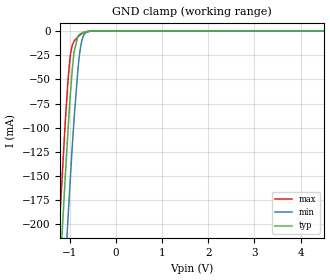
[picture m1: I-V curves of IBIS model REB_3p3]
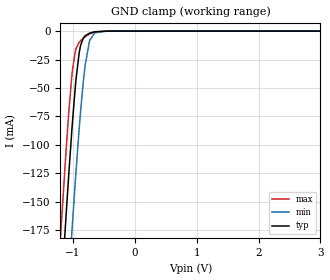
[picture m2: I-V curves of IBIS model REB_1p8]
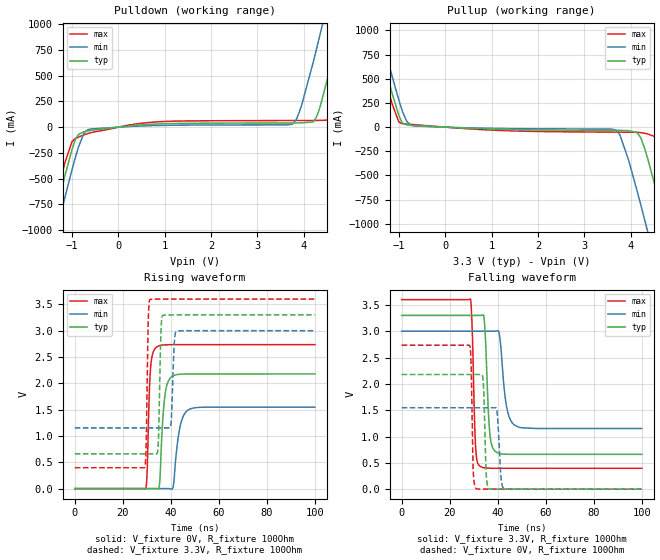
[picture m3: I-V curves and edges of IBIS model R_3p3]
|Texas Instruments Incorporated
| 3.3V RS-485 with flexible I/O supply and selectable speed
| Marketing part#   Digital Voltage Range   Package-type   #pins
| SN65HVD01   1.62V - 3.6V   VSON   10
[IBIS Ver]   4.1
[File name]   sn65hvd01.ibs
[File Rev]   1.1
[Date]   10/19/2016
[Source]
| Texas Instruments Incorporated.
| Analog-eLab Design Center, HPA
| 12500 TI Blvd
| Dallas, TX -75243
[Notes]   Revision History:
| Rev 1.2:10/19/2016
| - 2.5V model added for REB_xxx, R_xxx and DE_xxx.
|   Model names with a trailing _2p5 contains the model for
|   2.5V operation
| Rev 1.1: 04/09/2015
| - AB_ls model has been updated to better reflect the driver behavior.
| Rev 1.0: 05/08/2013
| - Initial version of the model
| - Model generated from simulations in TISPICE
| - C_comp although listed in numerical order of value are
|   obtained from varying PVT conditions. For PVT conditions for
|   each specific value refer the buffer description under
|   respective [Model]. IBIS model user is responsible for using
|   appropriate C_comp to simulate for Signal Integrity.
| - Warnings regarding combined Non-monotonicity of various models have been
|   reviewd and considered minor and can be ignored.
| - Model names with a trailing _1p8 contains the model for
|   1.8V operation.Model names with a trailing _3p3 contains the model
|   for 3.3V operation.
| - Mode names with a trailing _ls and _hs are for low speed and high speed
|   buffer operation, respectively.
[Disclaimer]
| This model is designed as an aid for customers of Texas Instruments.
| TI and its licensors and suppliers make no warranties, either expressed
| or implied, with respect to this  model, including the warranties of
| merchantability or fitness for a particular purpose. The model is
| provided solely on an "as is" basis. The entire risk as to its quality
| and performance is with the customer.
[Copyright]
 (C) Copyright 2013 Texas Instruments Incorporated.All rights reserved.
|   SN65HVD01
[Component]   SN65HVD01
[Manufacturer]   TI
[Package]   | 10 PIN VSON
|   typ   min   max
R_pkg   0.067   0.027   0.083
L_pkg   0.937nH   0.593nH   1.143nH
C_pkg   0.144pF   0.126pF   0.200pF
[Pin]  signal_name   model_name   R_pin   L_pin   C_pin
1   VL   POWER   NA   NA   NA
2   R   R   NA   NA   NA
3   DE   DE   NA   NA   NA
4   REB   REB   NA   NA   NA
5   D   REB   NA   NA   NA
6   GND   GND   NA   NA   NA
7   SLR   DE   NA   NA   NA
8   A   AB   NA   NA   NA
9   B   AB   NA   NA   NA
10   VCC   POWER   NA   NA   NA
[Diff Pin]  inv_pin  vdiff  tdelay_typ tdelay_min tdelay_max
8   9   200mV   NA   NA   NA
|   Model Selectors
[Model Selector]  DE
DE_3p3   DE buffer in 3.3V operation
DE_1p8   DE buffer in 1.8V operation
DE_2p5   DE buffer in 2.5V operation
[Model Selector]  REB
REB_3p3   REB buffer in 3.3V operation
REB_1p8   REB buffer in 1.8V operation
REB_2p5   REB buffer in 2.5V operation
[Model Selector]  R
R_3p3   R buffer in 3.3V operation
R_1p8   R buffer in 1.8V operation
R_2p5   R buffer in 2.5V operation
[Model Selector]  AB
AB_hs   high speed AB buffer operation
AB_ls   low speed AB buffer operation
| Models and submodels in the file (11): REB_3p3 (Input), REB_1p8 (Input), R_3p3 (Output), R_1p8 (Output), DE_3p3 (Input), DE_1p8 (Input), AB_ls (I/O), AB_hs (I/O), REB_2p5 (Input), R_2p5 (Output), DE_2p5 (Input)
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|   Model
[Model]   REB_3p3
Model_type   Input
Vinl = 0.99
Vinh = 2.31
|   typ   min   max
C_comp   0.767pF   0.735pF   0.817pF
[Voltage Range]   3.3   3   3.6
[Temperature Range]   27   125   -40
[Power Clamp Reference]   3.3   3   3.6
[GND Clamp Reference]   -0   -0   -0
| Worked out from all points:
|   GND clamp passes 1 mA (typ) near -0.68 V on its own axis
[GND Clamp]
|   Voltage   I(typ)   I(min)   I(max)
-3.3V     -2.277A    -2.364A    -2.225A
-1.231V   -268.8mA   -364.6mA   -209.6mA
-1.211V   -251mA     -346.7mA   -191.9mA
-1.092V   -147.7mA   -241.5mA   -91.49mA
-1.043V   -107.7mA   -199.2mA   -55.66mA
-983.4mV  -64.12mA   -150.4mA   -24.67mA
-914.1mV  -25.42mA   -97.58mA   -11.23mA
-815.1mV  -4.941mA   -36.43mA   -5.592mA
-726mV    -1.754mA   -8.002mA   -2.426mA
-656.7mV  -722uA     -1.89mA    -947.8uA
-498.3mV  -42.64uA   -89.28uA   -35.67uA
6.59V     0A         0A         0A
[POWER Clamp]
|   Voltage   I(typ)   I(min)   I(max)
-3.3V     0A         0A         0A
-3.28V    0A         0A         0A
-3.27V    0A         0A         0A
6.59V     0A         0A         0A
|   Model
[Model]   REB_1p8
Model_type   Input
Vinl = 0.54
Vinh = 1.26
|   typ   min   max
C_comp   0.767pF   0.735pF   0.817pF
[Voltage Range]   1.8   1.62   1.98
[Temperature Range]   27   125   -40
[Power Clamp Reference]   1.8   1.62   1.98
[GND Clamp Reference]   -0   -0   -0
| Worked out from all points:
|   GND clamp passes 1 mA (typ) near -0.67 V on its own axis
[GND Clamp]
|   Voltage   I(typ)   I(min)   I(max)
-1.8V     -806.5mA   -899.9mA   -749.6mA
-1.195V   -236.8mA   -332.4mA   -177.8mA
-1.109V   -161.6mA   -255.8mA   -104.5mA
-1.017V   -87.98mA   -177.7mA   -40.06mA
-963mV    -50.97mA   -134.3mA   -18.55mA
-898.2mV  -19.41mA   -86.34mA   -9.985mA
-871.2mV  -12.01mA   -68.3mA    -8.312mA
-801mV    -4.123mA   -29.96mA   -5.002mA
-725.4mV  -1.742mA   -7.906mA   -2.409mA
-644.4mV  -602.9uA   -1.468mA   -775.2uA
-450mV    -15.08uA   -36.58uA   -10.04uA
3.595V    0A         0A         0A
[POWER Clamp]
|   Voltage   I(typ)   I(min)   I(max)
-1.8V     0A         0A         0A
-1.789V   0A         0A         0A
-1.784V   0A         0A         0A
3.595V    0A         0A         0A
|   Model
[Model]   R_3p3
Model_type   Output
Polarity   Non-Inverting
Vmeas = 1.65
Vref = 0
Cref = 1pF
Rref = 100000
|   typ   min   max
C_comp   1.990pF   1.630pF   2.168pF
[Voltage Range]   3.3   3   3.6
[Temperature Range]   27   125   -40
[Pullup Reference]   3.3   3   3.6
[Pulldown Reference]   -0   -0   -0
[Power Clamp Reference]   3.3   3   3.6
[GND Clamp Reference]   -0   -0   -0
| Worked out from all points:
|   slope of the pulldown table from 0 to 0.495 V, typ, clamps not added: 22.9 ohm
|   slope of the pullup table from 0 to 0.495 V, typ, clamps not added: 43.1 ohm
|   falling waveform, V_fixture 3.3V, R_fixture 100Ohm: 20-80 % time 1.5ns typ, 2.46ns min, 1.12ns max; typ from 3.3 V to 0.661 V
|   rising waveform, V_fixture 0V, R_fixture 100Ohm: 20-80 % time 1.75ns typ, 2.57ns min, 1.12ns max; typ from 0 V to 2.18 V
|   rising waveform, V_fixture 3.3V, R_fixture 100Ohm: 20-80 % time 748ps typ, 872ps min, 662ps max; typ from 0.661 V to 3.3 V
|   falling waveform, V_fixture 0V, R_fixture 100Ohm: 20-80 % time 797ps typ, 1.09ns min, 671ps max; typ from 2.18 V to 0 V
[Pulldown]
|   Voltage   I(typ)   I(min)   I(max)
-3.3V     -4.044A    -4.245A    -3.921A
-1.722V   -1.54A     -1.752A    -1.41A
-1.29V    -719.7mA   -933.1mA   -588.4mA
-930mV    -125mA     -297.6mA   -111.2mA
-651mV    -36.01mA   -24.29mA   -60.9mA
3.768V    40.82mA    33.98mA    64.33mA
4.209V    52.95mA    638.1mA    64.93mA
4.362V    212.5mA    918.3mA    65.85mA
4.56V     551.6mA    1.29A      69.31mA
4.839V    1.073A     1.824A     404.5mA
5.019V    1.418A     2.172A     736.8mA
6.6V      4.507A     5.263A     3.811A
[Pullup]
|   Voltage   I(typ)   I(min)   I(max)
-3.3V     3.926A     4.09A      3.829A
-1.704V   1.389A     1.565A     1.282A
-1.218V   474.1mA    653.5mA    363.9mA
-948mV    62.52mA    198.9mA    37.75mA
-696mV    18.66mA    14.09mA    26.75mA
3.678V    -33.19mA   -30.63mA   -51.72mA
4.146V    -58.8mA    -668.9mA   -53.53mA
4.371V    -328.1mA   -1.084A    -71.12mA
4.632V    -796.9mA   -1.579A    -160.3mA
4.812V    -1.137A    -1.925A    -445.1mA
4.992V    -1.482A    -2.273A    -776.8mA
6.6V      -4.625A    -5.419A    -3.902A
[Ramp]
R_load = 100
|   typ   min   max
dV/dt_r   1.30679/1.7538e-09   0.928025/2.5712e-09   1.64055/1.11999e-09
dV/dt_f   1.58335/1.4976e-09   1.10814/2.45595e-09   1.922/1.12147e-09
[Falling Waveform]
V_fixture = 3.3V
V_fixture_min = 3V
V_fixture_max = 3.6V
R_fixture = 100Ohm
C_fixture = 0F
|   Time   V(typ)   V(min)   V(max)
0s        3.3V       3V         3.6V
28.66ns   3.3V       3V         3.611V
30.85ns   3.3V       3V         767.3mV
32.82ns   3.3V       3V         429.3mV
34.36ns   3.232V     3V         406.7mV
36.63ns   1.105V     3V         398.7mV
38.7ns    731.5mV    3V         397.2mV
40.59ns   679.8mV    2.965V     397.2mV
46.77ns   662mV      1.225V     397.1mV
100ns     661.1mV    1.153V     396.7mV
[Rising Waveform]
V_fixture = 0V
V_fixture_min = 0V
V_fixture_max = 0V
R_fixture = 100Ohm
C_fixture = 0F
|   Time   V(typ)   V(min)   V(max)
0s        983pV      30.98nV    480.2pV
29.53ns   89.04uV    116.2uV    -3.016mV
31.57ns   95.17uV    124.3uV    2.291V
34.34ns   -3.737mV   135.2uV    2.696V
35.39ns   133.5mV    139.3uV    2.716V
37.53ns   1.76V      147.7uV    2.729V
40.41ns   2.127V     -10.49mV   2.734V
43.73ns   2.171V     1.15V      2.734V
47.6ns    2.177V     1.503V     2.734V
100ns     2.178V     1.547V     2.734V
[Rising Waveform]
V_fixture = 3.3V
V_fixture_min = 3V
V_fixture_max = 3.6V
R_fixture = 100Ohm
C_fixture = 0F
|   Time   V(typ)   V(min)   V(max)
0s        661.1mV    1.153V     396.7mV
29.13ns   660.4mV    1.153V     405.9mV
30.59ns   660.4mV    1.153V     3.168V
31.26ns   660.4mV    1.153V     3.588V
34.61ns   747.4mV    1.153V     3.599V
35.84ns   2.908V     1.153V     3.599V
36.63ns   3.29V      1.153V     3.6V
39.96ns   3.298V     1.194V     3.6V
42.22ns   3.3V       2.986V     3.6V
100ns     3.3V       3V         3.6V
[Falling Waveform]
|Gnd
V_fixture = 0V
V_fixture_min = 0V
V_fixture_max = 0V
R_fixture = 100Ohm
C_fixture = 0F
|   Time   V(typ)   V(min)   V(max)
0s        2.178V     1.547V     2.734V
28.36ns   2.178V     1.547V     2.728V
29.82ns   2.178V     1.547V     348.9mV
31.1ns    2.178V     1.547V     7.742mV
33.79ns   2.117V     1.547V     867.9uV
35.2ns    301.4mV    1.547V     224.8uV
36.47ns   7.279mV    1.547V     220.4uV
39.6ns    1.1mV      1.508V     209.5uV
42.67ns   267.9uV    7.941mV    198.9uV
100ns     -149.8nV   639.4nV    -1.825nV
